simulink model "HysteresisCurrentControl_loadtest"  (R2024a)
settings: Solver=VariableStepAuto  StartTime=0.0  StopTime=1  FixedStep=1e-7  RelTol=1e-3
libraries: spsIGBTDiodeLib x6, spsThreePhaseSeriesRLCBranchLib x6, spsDiodeLib x6, spsGroundLib x4, spsThreePhaseBreakerLib x4, spsSeriesRLCBranchLib x3, spsThreePhaseVIMeasurementLib x3, spsMultimeterLib x3, spsThreePhaseSourceLib x2, spsTHDLib x2, spsPower3phInstantaneousLib x2, spsPVArrayLib x1

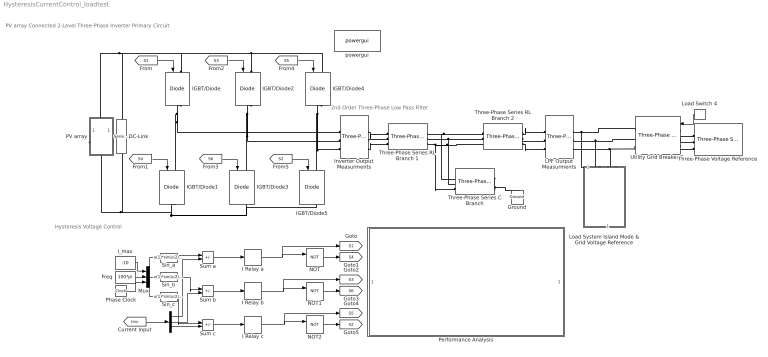
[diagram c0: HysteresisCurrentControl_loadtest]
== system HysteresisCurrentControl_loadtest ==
  note: 2nd Order Three-Phase Low Pass Filter
  note: PV array Connected 2-Level Three-Phase Inverter Primary Circuit
  note: Hysteresis Voltage Control
  DC-Link : spsSeriesRLCBranchLib/Series RLC Branch  LConnTagsString=__new0  RConnTagsString=__new0  BranchType=RC  Resistance=20e-3  Inductance=1e-3  SetiL0=off  InitialCurrent=0  Capacitance=81e-6  Setx0=off  InitialVoltage=0  Measurements=None
  Freq : Constant  Value=100*pi
  Ground : spsGroundLib/Ground  LConnTagsString=a
  I : Demux  Outputs=3
  I Relay a : Relay  OnSwitchValue=0.001  OffSwitchValue=-0.001
  I Relay b : Relay  OnSwitchValue=0.001  OffSwitchValue=-0.001
  I Relay c : Relay  OnSwitchValue=0.001  OffSwitchValue=-0.001
  IGBT/Diode{,1..5} (6 alike) : spsIGBTDiodeLib/IGBT//Diode  Ron=1e-3  Rs=1e5  Cs=inf  Measurements=off
  I_max : Constant  Value=-10
  Inverter Output Measurments : spsThreePhaseVIMeasurementLib/Three-Phase V-I Measurement  VoltageMeasurement=phase-to-phase  SetLabelV=on  LabelV=Vinv  Vpu=off  VpuLL=off  CurrentMeasurement=yes  SetLabelI=on  LabelI=Iinv  Ipu=off  Pbase=100e6  Vbase=500e3  OutputType=Complex  PhasorSimulation=off  PSBequivalent=0
  LPF Output Measurments : spsThreePhaseVIMeasurementLib/Three-Phase V-I Measurement  VoltageMeasurement=phase-to-phase  SetLabelV=on  LabelV=Vabc  Vpu=off  VpuLL=off  CurrentMeasurement=yes  SetLabelI=on  LabelI=Iabc  Ipu=off  Pbase=100e6  Vbase=500e3  OutputType=Complex  PhasorSimulation=off  PSBequivalent=0
  Load Switch 4 : DiscretePulseGenerator  PulseType=Time based  Period=1.2  PulseWidth=50  PhaseDelay=0.6
  Load System Island Mode & Grid Voltage Reference : Subsystem
  Mux : Mux  Inputs=3
  NOT : Logic  Operator=NOT  IconShape=distinctive  AllPortsSameDT=off  OutDataTypeStr=boolean
  NOT1 : Logic  Operator=NOT  IconShape=distinctive  AllPortsSameDT=off  OutDataTypeStr=boolean
  NOT2 : Logic  Operator=NOT  IconShape=distinctive  AllPortsSameDT=off  OutDataTypeStr=boolean
  PV array : Subsystem
  Performance Analysis : Subsystem
  Phase Clock : Clock
  Sin_a : Fcn  Expr=u(1)*sin(u(2)*u(3))
  Sin_b : Fcn  Expr=u(1)*sin(u(2)*u(3)-pi*2/3)
  Sin_c : Fcn  Expr=u(1)*sin(u(2)*u(3)+pi*2/3)
  Sum a : Sum  Inputs=|+-
  Sum b : Sum  Inputs=|+-
  Sum c : Sum  Inputs=|+-
  Three-Phase Series C Branch : spsThreePhaseSeriesRLCBranchLib/Three-Phase Series RLC Branch  LConnTagsString=A|B|C  RConnTagsString=A|B|C  BranchType=RC  Resistance=20e-3  Inductance=5.1e-5  Capacitance=81e-6  Measurements=None
  Three-Phase Series RL Branch 1 : spsThreePhaseSeriesRLCBranchLib/Three-Phase Series RLC Branch  LConnTagsString=A|B|C  RConnTagsString=A|B|C  BranchType=RL  Resistance=20e-3  Inductance=45e-6  Capacitance=1e-6  Measurements=None
  Three-Phase Series RL Branch 2 : spsThreePhaseSeriesRLCBranchLib/Three-Phase Series RLC Branch  LConnTagsString=A|B|C  RConnTagsString=A|B|C  BranchType=RL  Resistance=20e-3  Inductance=45e-6  Capacitance=1e-6  Measurements=None
  Three-Phase Voltage Reference : spsThreePhaseSourceLib/Three-Phase Source  InternalConnection=Yg  VoltagePhases=off  Voltage=240  PhaseAngle=60  Voltage_phases=[25e3 25e3 25e3]/sqrt(3)  PhaseAngles_phases=[0 -120 +120]  Frequency=50  NonIdealSource=on  SpecifyImpedance=off  Resistance=0.8929  Inductance=16.58e-3  ShortCircuitLevel=100e6  BaseVoltage=240  XRratio=7  BusType=swing  Pref=10e3  Qref=0  Prefabc=[10e3, 10e3, 10e3]  Qrefabc=[0, 0, 0]  Qmin=-inf  Qmax=inf
  Utility Grid Breaker 2 : spsThreePhaseBreakerLib/Three-Phase Breaker  InitialState=open  SwitchA=on  SwitchB=on  SwitchC=on  SwitchTimes="[1/60  5/60]"  External=on  BreakerResistance=0.01  SnubberResistance=1e6  SnubberCapacitance=inf  Measurements=None
  powergui : spspowerguiLib/powergui  Priority=1  SimulationMode=Discrete  SampleTime=1e-6  frequency=50  Iterations=50  frequencyindice=0  Pbase=100e6  ErrMax=1e-4  UnitsV=kV  UnitsW=MW  buscounter=0  FunctionMessages=off  echomessages=off  EnableUseOfTLC=off  CurrentSourceSwitches=off  DisableSnubberDevices=off  DisableRonSwitches=off  DisableVfSwitches=off  DisplayEquations=off  AutomaticDiscreteSolvers=off  SolverType=Tustin/Backward Euler (TBE)  Interpol=off  ExternalGateDelay=off  methode=off  Ts=100  x0status=blocks  SPID=on  SwTol=0  HookPort=off  NonlinearTolerance=1e-4  nMaxIteration=100  ContinueOnMaxIteration=off  RestoreLinks=warning  ResistiveCurrentMeasurement=off  Frange=[0:2:500]  Ylog=off  Xlog=on  ShowGrid=off  save=off  variable=ZData  structure=0  ZoomFFT=off  StartTime=0.0  cycles=1  DisplayStyle=1  fundamental=60  FreqAxis=off  MaxFrequency=1000  frequencyindicesteady=1  RmsSteady=1  display=off
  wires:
  NOT2/1 -> [S2]
  Sum b/1 -> I Relay b/1
  I Relay c/1 -> [S5], NOT2/1
  I Relay a/1 -> [S1], NOT/1
  Freq/1 -> Mux/2
  Sin_a/1 -> Sum a/1
  I_max/1 -> Mux/1
  Sin_c/1 -> Sum c/1
  Sin_b/1 -> Sum b/1
  Sum a/1 -> I Relay a/1
  I Relay b/1 -> [S3], NOT1/1
  Mux/1 -> Sin_a/1, Sin_c/1, Sin_b/1
  NOT1/1 -> [S6]
  I/2 -> Sum b/2
  Sum c/1 -> I Relay c/1
  [Iinv] -> I/1
  [S2] -> IGBT/Diode5/1
  [S3] -> IGBT/Diode2/1
  [S1] -> IGBT/Diode/1
  [S4] -> IGBT/Diode1/1
  Phase Clock/1 -> Mux/3
  [S6] -> IGBT/Diode3/1
  I/1 -> Sum a/2
  NOT/1 -> [S4]
  [S5] -> IGBT/Diode4/1
  I/3 -> Sum c/2
  Load Switch 4/1 -> Utility Grid Breaker 2/1
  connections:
  IGBT/Diode1/RConn1 -- DC-Link/RConn1 -- PV array/RConn1 -- IGBT/Diode5/RConn1 -- IGBT/Diode3/RConn1
  IGBT/Diode2/RConn1 -- IGBT/Diode3/LConn1 -- Inverter Output Measurments/LConn2
  Three-Phase Series RL Branch 2/LConn1 -- Three-Phase Series C Branch/LConn1 -- Three-Phase Series RL Branch 1/RConn1
  Three-Phase Series RL Branch 1/RConn3 -- Three-Phase Series RL Branch 2/LConn3 -- Three-Phase Series C Branch/LConn3
  Three-Phase Series RL Branch 2/LConn2 -- Three-Phase Series C Branch/LConn2 -- Three-Phase Series RL Branch 1/RConn2
  IGBT/Diode2/LConn1 -- DC-Link/LConn1 -- PV array/LConn1 -- IGBT/Diode/LConn1 -- IGBT/Diode4/LConn1
  IGBT/Diode/RConn1 -- IGBT/Diode1/LConn1 -- Inverter Output Measurments/LConn1
  IGBT/Diode4/RConn1 -- IGBT/Diode5/LConn1 -- Inverter Output Measurments/LConn3
  Three-Phase Series RL Branch 2/RConn3 -- LPF Output Measurments/LConn3
  Inverter Output Measurments/RConn1 -- Three-Phase Series RL Branch 1/LConn1
  Inverter Output Measurments/RConn2 -- Three-Phase Series RL Branch 1/LConn2
  Three-Phase Series RL Branch 2/RConn2 -- LPF Output Measurments/LConn2
  Inverter Output Measurments/RConn3 -- Three-Phase Series RL Branch 1/LConn3
  Three-Phase Series RL Branch 2/RConn1 -- LPF Output Measurments/LConn1
  LPF Output Measurments/RConn1 -- Utility Grid Breaker 2/RConn1 -- Load System Island Mode & Grid Voltage Reference/LConn1
  LPF Output Measurments/RConn2 -- Utility Grid Breaker 2/RConn2 -- Load System Island Mode & Grid Voltage Reference/LConn2
  LPF Output Measurments/RConn3 -- Utility Grid Breaker 2/RConn3 -- Load System Island Mode & Grid Voltage Reference/LConn3
  Utility Grid Breaker 2/LConn2 -- Three-Phase Voltage Reference/RConn2
  Utility Grid Breaker 2/LConn1 -- Three-Phase Voltage Reference/RConn1
  Utility Grid Breaker 2/LConn3 -- Three-Phase Voltage Reference/RConn3
  Three-Phase Series C Branch/RConn1 -- Three-Phase Series C Branch/RConn2 -- Ground/LConn1 -- Three-Phase Series C Branch/RConn3

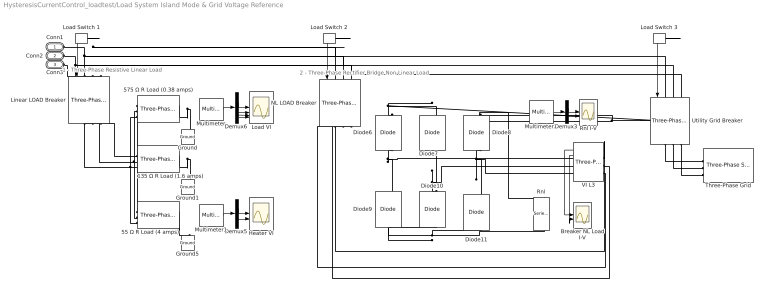
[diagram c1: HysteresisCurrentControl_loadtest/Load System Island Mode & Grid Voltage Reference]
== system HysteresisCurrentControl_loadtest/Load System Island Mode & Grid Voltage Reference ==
  note: 1 - Three-Phase Resistive Linear Load
  note: 2 - Three-Phase Rectifier Bridge Non-Linear Load
  135 Ω R Load (1.6 amps) : spsThreePhaseSeriesRLCBranchLib/Three-Phase Series RLC Branch  LConnTagsString=A|B|C  RConnTagsString=A|B|C  BranchType=R  Resistance=135  Inductance=5.1e-3  Capacitance=1e-6  Measurements=Branch voltages and currents
  55 Ω R Load (4 amps) : spsThreePhaseSeriesRLCBranchLib/Three-Phase Series RLC Branch  LConnTagsString=A|B|C  RConnTagsString=A|B|C  BranchType=R  Resistance=55  Inductance=5.1e-3  Capacitance=1e-6  Measurements=Branch voltages and currents
  575 Ω R Load (0.38 amps) : spsThreePhaseSeriesRLCBranchLib/Three-Phase Series RLC Branch  LConnTagsString=A|B|C  RConnTagsString=A|B|C  BranchType=R  Resistance=575  Inductance=5.1e-3  Capacitance=1e-6  Measurements=Branch voltages and currents
  Breaker NL Load I-V : Scope  NumInputPorts=2
  Demux3 : Demux  Outputs=2
  Demux5 : Demux  Outputs=2
  Demux6 : Demux
  Diode{6..11} (6 alike) : spsDiodeLib/Diode  Ron=0.001  Lon=0  Vf=0.8  IC=0  UseSnubber=0  Rs=10e+6  Cs=250e-9  Measurements=off
  Ground : spsGroundLib/Ground  LConnTagsString=a
  Ground1 : spsGroundLib/Ground  LConnTagsString=a
  Ground5 : spsGroundLib/Ground  LConnTagsString=a
  Heater VI : Scope  NumInputPorts=2
  Linear LOAD Breaker : spsThreePhaseBreakerLib/Three-Phase Breaker  InitialState=open  SwitchA=on  SwitchB=on  SwitchC=on  SwitchTimes="[1/60  5/60]"  External=on  BreakerResistance=0.01  SnubberResistance=1e6  SnubberCapacitance=inf  Measurements=None
  Load Switch 1 : DiscretePulseGenerator  PulseType=Time based  Period=0.6  PulseWidth=100/3
  Load Switch 2 : DiscretePulseGenerator  PulseType=Time based  Period=0.6  PulseWidth=100/3  PhaseDelay=0.2
  Load Switch 3 : DiscretePulseGenerator  PulseType=Time based  Period=0.6  PulseWidth=100/3  PhaseDelay=0.4
  Load VI : Scope  NumInputPorts=4
  Multimeter : spsMultimeterLib/Multimeter  L=20  sel=[8 2 18 12]  yselected={}  Gain=[1 1 1 1]  OutputType=Complex  PlotAtSimulationStop=off  PhasorSimulation=off
  Multimeter1 : spsMultimeterLib/Multimeter  L=20  sel=[5 15]  yselected={}  Gain=[1 1]  OutputType=Complex  PlotAtSimulationStop=off  PhasorSimulation=off
  Multimeter2 : spsMultimeterLib/Multimeter  L=20  sel=[1 11]  yselected={}  Gain=[1 1]  OutputType=Complex  PlotAtSimulationStop=off  PhasorSimulation=off
  NL LOAD Breaker : spsThreePhaseBreakerLib/Three-Phase Breaker  InitialState=open  SwitchA=on  SwitchB=on  SwitchC=on  SwitchTimes="[1/60  5/60]"  External=on  BreakerResistance=0.01  SnubberResistance=1e6  SnubberCapacitance=inf  Measurements=None
  Rnl : spsSeriesRLCBranchLib/Series RLC Branch  LConnTagsString=__new0  RConnTagsString=__new0  BranchType=R  Resistance=1000  Inductance=1e-6  SetiL0=off  InitialCurrent=0  Capacitance=0.01598  Setx0=off  InitialVoltage=0  Measurements=Branch voltage and current
  Rnl I-V : Scope  NumInputPorts=2
  Three-Phase Grid : spsThreePhaseSourceLib/Three-Phase Source  InternalConnection=Yg  VoltagePhases=off  Voltage=240  PhaseAngle=0  Voltage_phases=[25e3 25e3 25e3]/sqrt(3)  PhaseAngles_phases=[0 -120 +120]  Frequency=50  NonIdealSource=on  SpecifyImpedance=off  Resistance=0.8929  Inductance=16.58e-3  ShortCircuitLevel=100e6  BaseVoltage=240  XRratio=7  BusType=swing  Pref=10e3  Qref=0  Prefabc=[10e3, 10e3, 10e3]  Qrefabc=[0, 0, 0]  Qmin=-inf  Qmax=inf
  Utility Grid Breaker : spsThreePhaseBreakerLib/Three-Phase Breaker  InitialState=open  SwitchA=on  SwitchB=on  SwitchC=on  SwitchTimes="[1/60  5/60]"  External=on  BreakerResistance=0.01  SnubberResistance=1e6  SnubberCapacitance=inf  Measurements=None
  VI L3 : spsThreePhaseVIMeasurementLib/Three-Phase V-I Measurement  VoltageMeasurement=phase-to-phase  SetLabelV=off  LabelV=Vabc  Vpu=off  VpuLL=off  CurrentMeasurement=yes  SetLabelI=off  LabelI=Iabc  Ipu=off  Pbase=100e6  Vbase=500e3  OutputType=Complex  PhasorSimulation=off  PSBequivalent=0
  Conn1 : PMIOPort  Side=Left
  Conn2 : PMIOPort  Port=2  Side=Left
  Conn3 : PMIOPort  Port=3  Side=Left
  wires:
  Demux5/2 -> Heater VI/2
  Demux6/2 -> Load VI/2
  Demux6/4 -> Load VI/4
  Demux6/1 -> Load VI/1
  Multimeter/1 -> Demux6/1
  Demux6/3 -> Load VI/3
  Demux5/1 -> Heater VI/1
  Multimeter1/1 -> Demux5/1
  Load Switch 1/1 -> Linear LOAD Breaker/1
  Load Switch 2/1 -> NL LOAD Breaker/1
  Load Switch 3/1 -> Utility Grid Breaker/1
  Multimeter2/1 -> Demux3/1
  Demux3/1 -> Rnl I-V/1
  Demux3/2 -> Rnl I-V/2
  VI L3/2 -> Breaker NL Load I-V/2
  VI L3/1 -> Breaker NL Load I-V/1
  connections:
  55 Ω R Load (4 amps)/LConn2 -- 135 Ω R Load (1.6 amps)/LConn2 -- Linear LOAD Breaker/RConn2 -- 575 Ω R Load (0.38 amps)/LConn2
  55 Ω R Load (4 amps)/LConn3 -- 135 Ω R Load (1.6 amps)/LConn3 -- Linear LOAD Breaker/RConn3 -- 575 Ω R Load (0.38 amps)/LConn3
  55 Ω R Load (4 amps)/RConn1 -- 55 Ω R Load (4 amps)/RConn2 -- 55 Ω R Load (4 amps)/RConn3 -- Ground5/LConn1
  55 Ω R Load (4 amps)/LConn1 -- 135 Ω R Load (1.6 amps)/LConn1 -- Linear LOAD Breaker/RConn1 -- 575 Ω R Load (0.38 amps)/LConn1
  575 Ω R Load (0.38 amps)/RConn1 -- Ground/LConn1 -- 575 Ω R Load (0.38 amps)/RConn3 -- 575 Ω R Load (0.38 amps)/RConn2
  135 Ω R Load (1.6 amps)/RConn1 -- Ground1/LConn1 -- 135 Ω R Load (1.6 amps)/RConn3 -- 135 Ω R Load (1.6 amps)/RConn2
  Utility Grid Breaker/RConn1 -- Three-Phase Grid/RConn1
  Utility Grid Breaker/RConn3 -- Three-Phase Grid/RConn3
  Utility Grid Breaker/RConn2 -- Three-Phase Grid/RConn2
  Conn1/RConn1 -- NL LOAD Breaker/LConn1 -- Utility Grid Breaker/LConn1 -- Linear LOAD Breaker/LConn1
  Conn2/RConn1 -- NL LOAD Breaker/LConn2 -- Utility Grid Breaker/LConn2 -- Linear LOAD Breaker/LConn2
  Conn3/RConn1 -- NL LOAD Breaker/LConn3 -- Utility Grid Breaker/LConn3 -- Linear LOAD Breaker/LConn3
  Diode6/RConn1 -- Rnl/LConn1 -- Diode8/RConn1 -- Diode7/RConn1
  Diode6/LConn1 -- Diode9/RConn1 -- VI L3/RConn1
  Diode8/LConn1 -- Diode11/RConn1 -- VI L3/RConn3
  Diode9/LConn1 -- Rnl/RConn1 -- Diode11/LConn1 -- Diode10/LConn1
  Diode10/RConn1 -- Diode7/LConn1 -- VI L3/RConn2
  NL LOAD Breaker/RConn1 -- VI L3/LConn1
  VI L3/LConn2 -- NL LOAD Breaker/RConn2
  VI L3/LConn3 -- NL LOAD Breaker/RConn3

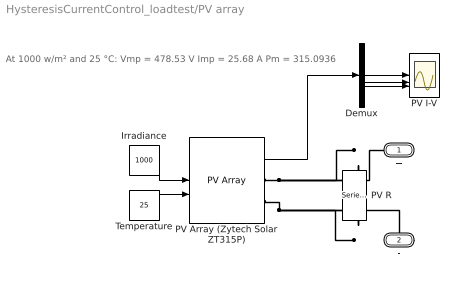
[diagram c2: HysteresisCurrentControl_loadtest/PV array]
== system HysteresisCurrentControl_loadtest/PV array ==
  note: At 1000 w/m² and 25 °C: Vmp = 478.53 V Imp = 25.68 A Pm = 315.0936
  Demux : Demux  Outputs=5
  Irradiance : Constant  Value=1000
  PV I-V : Scope  NumInputPorts=5
  PV Array (Zytech Solar ZT315P) : spsPVArrayLib/PV Array  Npar=3  Nser=13  PlotType=array @ 25 deg.C & specified irradiances  S_vec="[ 1000  500  100 ]"  Temp_C_vec="[ 45 25  ]"  ModuleName=Zytech Solar ZT315P  PlotWhenSelected=off  Pm=315.0936  Ncell=72  Voc=46.44  Isc=9.01  Vm=36.81  Im=8.56  beta_Voc_pc=-0.3199  alpha_Isc_pc=0.048302  beta_Voc=-0.14856  alpha_Isc=0.004352  IL=9.0792  I0=6.901e-11  nI=0.9809  Rsh=572.7811  Rs=0.50125  RobustModel=off  RobustCellTemperature=313.3991  BAL=on  Tc=1e-6  Tfilter=5e-5
  PV R : spsSeriesRLCBranchLib/Series RLC Branch  LConnTagsString=__new0  RConnTagsString=__new0  BranchType=R  Resistance=18.6  Inductance=1e-3  SetiL0=off  InitialCurrent=0  Capacitance=1e-6  Setx0=off  InitialVoltage=0  Measurements=None
  Temperature : Constant  Value=25
  + : PMIOPort  Side=Left
  - : PMIOPort  Port=2  Side=Right
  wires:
  PV Array (Zytech Solar ZT315P)/1 -> Demux/1
  Demux/3 -> PV I-V/3
  Temperature/1 -> PV Array (Zytech Solar ZT315P)/2
  Demux/2 -> PV I-V/2
  Irradiance/1 -> PV Array (Zytech Solar ZT315P)/1
  Demux/1 -> PV I-V/1
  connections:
  PV Array (Zytech Solar ZT315P)/RConn1 -- PV R/LConn1 -- +/RConn1
  PV Array (Zytech Solar ZT315P)/RConn2 -- PV R/RConn1 -- -/RConn1

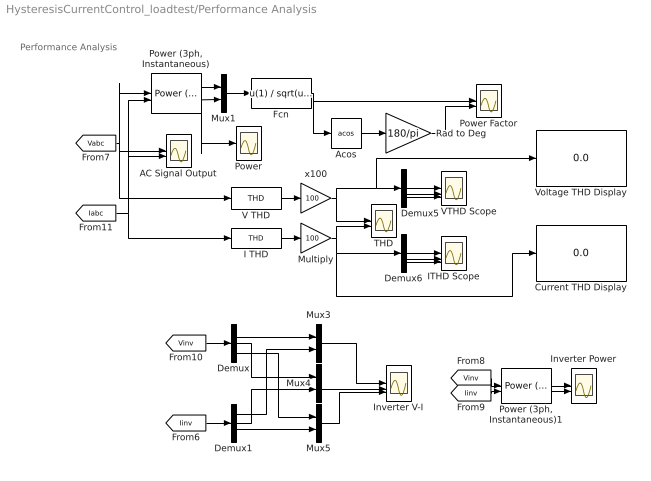
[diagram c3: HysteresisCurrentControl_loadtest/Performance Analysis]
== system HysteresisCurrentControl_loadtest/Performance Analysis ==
  note: Performance Analysis
  AC Signal Output : Scope  NumInputPorts=2
  Acos : Trigonometry  Operator=acos
  Current THD Display : Display
  Demux{,1,5..6} (4 alike) : Demux  Outputs=3
  Fcn : Fcn  Expr=u(1) / sqrt(u(1)^2 + u(2)^2)
  I THD : spsTHDLib/THD  Freq=50  Ts=0
  ITHD Scope : Scope  NumInputPorts=3
  Inverter V-I : Scope  NumInputPorts=3
  Inverter Power : Scope  NumInputPorts=2
  Multiply : Gain  Gain=100
  Mux{1,3..5} (4 alike) : Mux  Inputs=2
  Power : Scope
  "Power (3ph, Instantaneous)" : spsPower3phInstantaneousLib/Power (3ph, Instantaneous)
  "Power (3ph, Instantaneous)1" : spsPower3phInstantaneousLib/Power (3ph, Instantaneous)
  Power Factor : Scope  NumInputPorts=2
  Rad to Deg : Gain  Gain=180/pi
  THD : Scope  NumInputPorts=2
  V THD : spsTHDLib/THD  Freq=50  Ts=0
  VTHD Scope : Scope  NumInputPorts=3
  Voltage THD Display : Display
  x100 : Gain  Gain=100
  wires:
  x100/1 -> THD/1, Voltage THD Display/1, Demux5/1
  Fcn/1 -> Power Factor/1, Acos/1
  Demux5/2 -> VTHD Scope/2
  [Iabc] -> I THD/1, "Power (3ph, Instantaneous)"/2, AC Signal Output/2
  Demux6/3 -> ITHD Scope/3
  "Power (3ph, Instantaneous)"/1 -> Power/1, Mux1/1
  Demux6/2 -> ITHD Scope/2
  Multiply/1 -> Current THD Display/1, Demux6/1, THD/2
  Demux5/1 -> VTHD Scope/1
  Rad to Deg/1 -> Power Factor/2
  V THD/1 -> x100/1
  I THD/1 -> Multiply/1
  Demux5/3 -> VTHD Scope/3
  [Vabc] -> V THD/1, AC Signal Output/1, "Power (3ph, Instantaneous)"/1
  "Power (3ph, Instantaneous)"/2 -> Mux1/2
  Acos/1 -> Rad to Deg/1
  Mux1/1 -> Fcn/1
  Demux6/1 -> ITHD Scope/1
  Demux/3 -> Mux5/1
  "Power (3ph, Instantaneous)1"/2 -> Inverter Power/2
  Demux1/2 -> Mux4/2
  Demux/2 -> Mux4/1
  Mux5/1 -> Inverter V-I/3
  Demux1/3 -> Mux5/2
  [Vinv] -> "Power (3ph, Instantaneous)1"/1
  Mux3/1 -> Inverter V-I/1
  [Iinv] -> Demux1/1
  Demux1/1 -> Mux3/2
  [Iinv] -> "Power (3ph, Instantaneous)1"/2
  [Vinv] -> Demux/1
  "Power (3ph, Instantaneous)1"/1 -> Inverter Power/1
  Mux4/1 -> Inverter V-I/2
  Demux/1 -> Mux3/1
